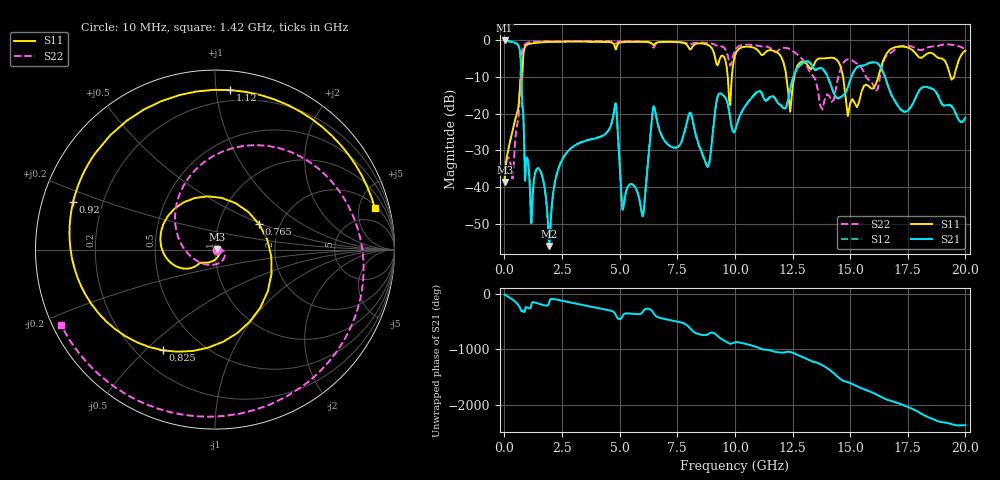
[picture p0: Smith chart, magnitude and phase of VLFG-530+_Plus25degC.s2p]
! Mini-Circuits
! S2P DATA File Format
! Type: LOW PASS FILTER
! Model: VLFG-530+
! All S Parameters are in dB deg format
! TEST CONDITIONS: INPUT POWER = 0 dBm @ Temperature = +25 deg C
# MHz S dB R 50
!Frequency  S11 dB  S11 DEG  S21 dB  S21 DEG  S12 dB  S12 DEG  S22 dB  S22 DEG
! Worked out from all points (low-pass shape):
!   652 points, 10 MHz to 20 GHz, reference 50 ohm
!   highest |S21| = -0.11 dB at 11 MHz (marker M1); lowest = -56.0 dB at 1.94 GHz (marker M2)
!   |S21| within 3 dB of the highest: start of sweep to 676.6 MHz
!   lowest |S11| = -38.6 dB at 12 MHz (marker M3), VSWR 1.02, Z = 51.2 + j0.124 ohm
!   |S11| at or under -10 dB: start of sweep to 714.7 MHz; 12.23 GHz to 12.58 GHz (344.8 MHz wide, 2.78 % of centre); 14.69 GHz to 16.22 GHz (1.529 GHz wide, 9.89 % of centre)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
!   |S22| runs from -38.6 to -0.2 dB; largest |S21 - S12| = 0.012
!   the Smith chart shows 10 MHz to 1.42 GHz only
!   S11 on the Smith chart (normalised r, x): 10 MHz: 1.02, +0.00; 765 MHz: 1.56, +0.48; 825 MHz: 0.30, -0.57; 920 MHz: 0.09, +0.16; 1.12 GHz: 0.12, +1.09; 1.42 GHz: 2.32, +7.04
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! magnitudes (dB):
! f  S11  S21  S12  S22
! 10 MHz  -38.3  -0.1  -0.1  -38.2
! 11 MHz  -38.5  -0.1  -0.1  -38.6
! 12 MHz  -38.6  -0.1  -0.1  -38.5
! 365 MHz  -24.4  -0.5  -0.5  -37.7
! 765 MHz  -10.9  -16.1  -16.1  -3.2
! 825 MHz  -4.0  -21.0  -21.0  -1.8
! 920 MHz  -1.6  -35.5  -35.5  -1.0
! 1.12 GHz  -1.0  -42.0  -42.0  -0.6
! 1.42 GHz  -0.7  -35.0  -35.0  -0.4
! 1.94 GHz  -0.5  -56.0  -56.0  -0.3
! 2.36 GHz  -0.4  -34.7  -34.7  -0.3
! 3.35 GHz  -0.4  -27.8  -27.7  -0.2
! 4.8 GHz  -2.0  -17.7  -17.6  -0.8
! 5.125 GHz  -0.6  -46.1  -46.1  -0.3
! 6 GHz  -0.5  -47.9  -47.9  -0.4
! 6.45 GHz  -1.3  -18.7  -18.6  -2.0
! 6.675 GHz  -0.6  -23.4  -23.3  -0.7
! 10.05 GHz  -3.5  -23.7  -23.8  -2.4
! 13.4 GHz  -7.2  -7.6  -7.7  -9.8
! 15.1 GHz  -16.1  -9.3  -9.3  -5.6
! 16.7 GHz  -2.8  -13.5  -13.6  -3.6
! 20 GHz  -2.8  -21.1  -21.1  -2.6
